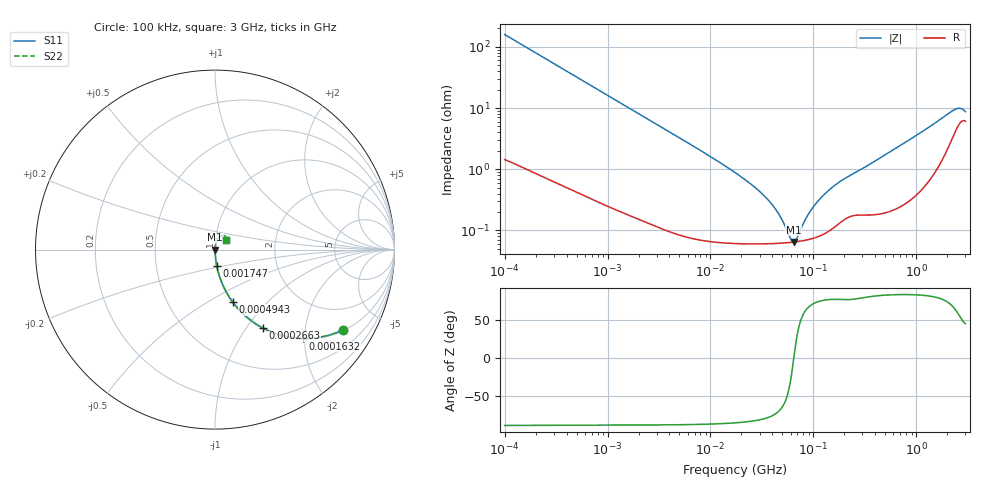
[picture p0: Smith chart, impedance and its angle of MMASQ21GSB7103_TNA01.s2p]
! MMASQ21GSB7103_TNA01  S-PARAMETER MODEL  ( Standard Model )
! Model Generated by TAIYO YUDEN Corporation (http://www.ty-top.com)
! Version 1.0
! TAIYO YUDEN Control No. 220601
! Copyright(c) 2013 TAIYO YUDEN CO.,LTD. All Rights Reserved.
! Product Description (link to TY-COMPAS)
! https://ds.yuden.co.jp/TYCOMPAS/or/detail?pn=MMASQ21GSB7103KTNA01&u=M
! Products Name : Multilayer Ceramic Capacitors
! Characteristics :
!  Capacitance : 0.01 [uF] , Rated Voltage : 250 [V] , TCC : X7R
!  Case Size : 2.0 x 1.25 / 0.079 x 0.049 [mm/inch] , Thickness : 1.25 / 0.049 [mm/inch]
!  (Conditions: Temperature = 25 [degC] , DC Bias Voltage = 0 [V])
! External Node Assignments :
!  1  o---| |---o  2
! GND o---------o GND
! Frequency Range : 100kHz  -  3GHz  [ 401 STEP ]
# MHZ S RI R 50
! Freq[MHz].  S11 Real  S11 Imag  S21 Real  S21 Imag  S12 Real  S12 Imag  S22 Real  S22 Imag
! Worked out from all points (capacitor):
!   401 points, 100 kHz to 3 GHz, reference 50 ohm
!   read as one part in series: C = 9.98 nF near 105.3 kHz
!   lowest |Z| = 64.4 mohm at 64.48 MHz (marker M1)
!   series resonance near 64.54 MHz, so ESL is about 610 pH
!   S11 on the Smith chart (normalised r, x): 100 kHz: 1.03, -3.18; 163.2 kHz: 1.02, -1.96; 266.3 kHz: 1.01, -1.20; 494.3 kHz: 1.01, -0.65; 1.747 MHz: 1.00, -0.19; 3 GHz: 1.12, +0.12
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0.1  0.7152 -0.4468  0.2848 0.4468  0.2848 0.4468  0.7152 -0.4468
0.163179  0.4892 -0.4948  0.5108 0.4948  0.5108 0.4948  0.4892 -0.4948
0.266273  0.268 -0.4373  0.732 0.4373  0.732 0.4373  0.268 -0.4373
0.494258  0.0989 -0.2921  0.9011 0.2921  0.9011 0.2921  0.0989 -0.2921
0.562235  0.0788 -0.2629  0.9212 0.2629  0.9212 0.2629  0.0788 -0.2629
1.747435  0.0102 -0.0919  0.9898 0.0919  0.9898 0.0919  0.0102 -0.0919
3.161081  0.00375 -0.0513  0.9962 0.0513  0.9962 0.0513  0.00375 -0.0513
17.7727  0.000681 -0.00854  0.9993 0.00854  0.9993 0.00854  0.000681 -0.00854
28.26337  0.000623 -0.0047  0.9994 0.0047  0.9994 0.0047  0.000623 -0.0047
38.50681  0.000614 -0.00275  0.9994 0.00275  0.9994 0.00275  0.000614 -0.00275
47.32384  0.000619 -0.00161  0.9994 0.00161  0.9994 0.00161  0.000619 -0.00161
59.67813  0.000635 -0.0004  0.9994 0.0004  0.9994 0.0004  0.000635 -0.0004
64.47533  0.000644 -5.02e-06  0.9994 5.02e-06  0.9994 5.02e-06  0.000644 -5.02e-06
69.65816  0.000655 0.00039  0.9993 -0.00039  0.9993 -0.00039  0.000655 0.00039
83.42988  0.000691 0.00132  0.9993 -0.00132  0.9993 -0.00132  0.000691 0.00132
97.38194  0.000738 0.00216  0.9993 -0.00216  0.9993 -0.00216  0.000738 0.00216
126.0104  0.000881 0.00368  0.9991 -0.00368  0.9991 -0.00368  0.000881 0.00368
171.6802  0.00127 0.00574  0.9987 -0.00574  0.9987 -0.00574  0.00127 0.00574
547.5153  0.00237 0.0187  0.9976 -0.0187  0.9976 -0.0187  0.00237 0.0187
2259.438  0.0384 0.0783  0.9616 -0.0783  0.9616 -0.0783  0.0384 0.0783
2637.286  0.0584 0.0729  0.9416 -0.0729  0.9416 -0.0729  0.0584 0.0729
3000  0.0606 0.0552  0.9394 -0.0552  0.9394 -0.0552  0.0606 0.0552
